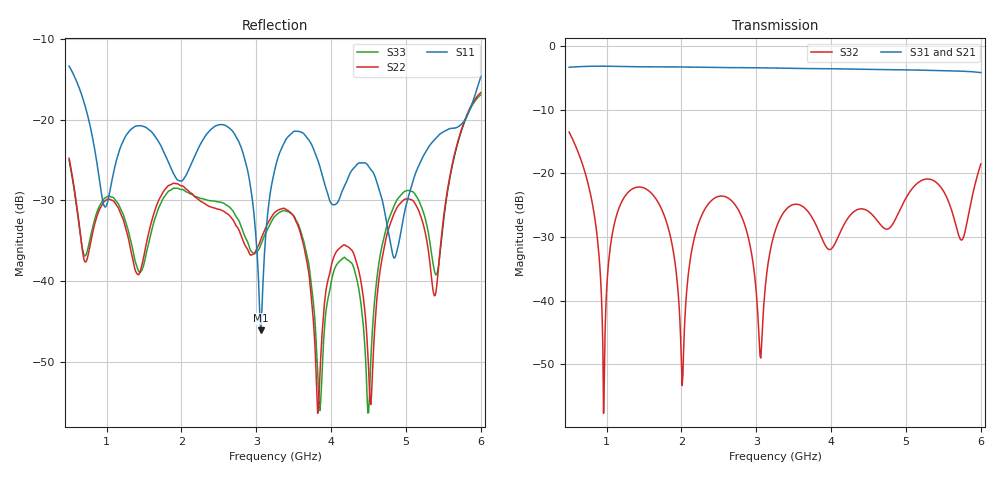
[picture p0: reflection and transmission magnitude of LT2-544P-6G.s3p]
! MTS Systemtechnik GmbH
! S-Parameters
! Model: LT2-544P-6G
! Rohde & Schwarz ZVB8 2Ports - Version 3.20 - 1145.1010k08 SN: 100119
! Converted & adapted with MATLAB
!		|  MTS  |
!		|  |--o OUT 2 (Port 3)
! C (Port 1) o--| LT2-544P-6G |
!		|  |--o OUT 1 (Port 2)
! S3P File: Measurements:
! <S11,S12,S13>,
! <S21,S22,S23>,
! <S31,S32,S33>:
# HZ  S  DB  R  50.00
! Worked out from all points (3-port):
!   551 points, 500 MHz to 6 GHz, reference 50 ohm
!   strongest paths, dB at 500 MHz, 1.87 GHz, 3.25 GHz, 4.63 GHz, 6 GHz:
!     S31: -3.3, -3.3, -3.4, -3.7, -4.2
!     S21: -3.3, -3.3, -3.5, -3.7, -4.1
!     S32: -13.5, -30.8, -29.1, -27.6, -18.5
!   lowest |S11| = -46.1 dB at 3.06 GHz (marker M1), VSWR 1.01, Z = 50.5 - j0.101 ohm
!   |S11| at or under -10 dB: start of sweep to end of sweep
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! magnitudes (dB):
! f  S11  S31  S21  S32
! 500 MHz  -13.4  -3.3  -3.3  -13.5
! 960 MHz  -30.5  -3.1  -3.2  -57.7
! 1.42 GHz  -20.8  -3.2  -3.2  -22.1
! 2.01 GHz  -27.6  -3.3  -3.3  -53.3
! 2.5 GHz  -20.6  -3.4  -3.4  -23.6
! 3.06 GHz  -46.1  -3.4  -3.4  -49.0
! 3.25 GHz  -26.1  -3.4  -3.5  -29.1
! 4.5 GHz  -25.8  -3.6  -3.6  -26.0
! 4.77 GHz  -34.2  -3.7  -3.7  -28.7
! 6 GHz  -14.6  -4.2  -4.1  -18.5
